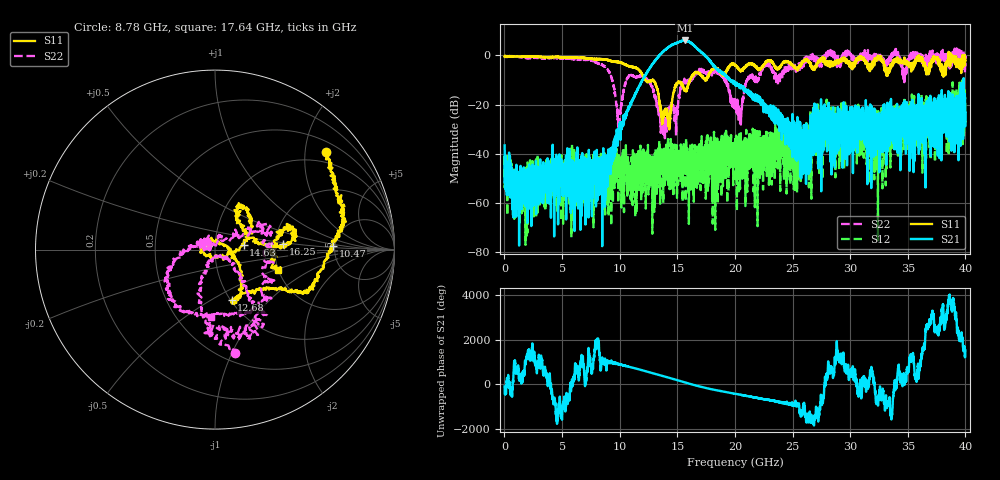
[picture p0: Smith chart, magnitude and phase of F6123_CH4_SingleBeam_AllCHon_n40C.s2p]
!Keysight Technologies,N5245B,MY55451909,A.17.20.08
!Date: Tuesday, November 21, 2023 17:28:04
!Correction: S11(C  2-Port  )
!S21(C  2-Port  )
!S12(C  2-Port  )
!S22(C  2-Port  )
!S2P File: Measurements: S11, S21, S12, S22:
# Hz S  RI  R 50
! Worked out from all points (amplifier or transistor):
!   4000 points, 10 MHz to 40 GHz, reference 50 ohm
!   highest |S21| = 6.1 dB at 15.64 GHz (marker M1)
!   |S21| within 3 dB of that: 14.18 GHz to 16.65 GHz (2.468 GHz wide, 16 % of centre)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
!   unconditionally stable (mu >= 1): start of sweep to 26.54 GHz; 26.75 GHz to 27.77 GHz; 32.61 GHz to 33.59 GHz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
!   at 6.67 GHz: K = 1996.61, MAG = -36.6 dB, |S12| = -46.4 dB
!   at 20.01 GHz: K = 145.94, MAG = -9.1 dB, |S12| = -42.6 dB
!   at 40 GHz: K = 23.65, MAG = -16.5 dB, |S12| = -23.7 dB
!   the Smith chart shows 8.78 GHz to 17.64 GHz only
!   S11 on the Smith chart (normalised r, x): 8.78 GHz: 0.74, +2.47; 10.47 GHz: 4.82, +0.38; 12.68 GHz: 1.01, -0.62; 14.63 GHz: 1.38, +0.08; 16.25 GHz: 2.21, +0.15; 17.64 GHz: 2.00, -0.53
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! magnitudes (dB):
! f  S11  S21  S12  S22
! 10 MHz  -0.4  -36.6  -41.1  -0.5
! 860 MHz  -0.4  -58.6  -62.6  -0.4
! 6.68 GHz  -0.9  -40.8  -46.9  -1.7
! 8.78 GHz  -1.7  -57.1  -48.1  -4.6
! 9.89 GHz  -2.7  -30.0  -42.7  -29.1
! 10.47 GHz  -3.6  -25.7  -45.9  -11.9
! 12.68 GHz  -10.6  -4.8  -47.5  -11.7
! 13.34 GHz  -15.3  -0.6  -45.5  -20.8
! 14.22 GHz  -28.8  3.3  -53.5  -25.8
! 14.63 GHz  -15.8  4.4  -48.0  -20.1
! 15.64 GHz  -13.9  6.1  -47.4  -9.8
! 16.25 GHz  -8.4  4.8  -43.0  -9.1
! 17.64 GHz  -8.6  -1.2  -42.1  -8.5
! 20.01 GHz  -3.8  -11.5  -42.6  -18.1
! 20.44 GHz  -6.1  -12.4  -54.4  -27.5
! 21.11 GHz  -3.7  -15.2  -43.6  -9.7
! 22.65 GHz  -2.8  -20.4  -36.0  -3.3
! 23.73 GHz  -4.9  -28.1  -46.0  -11.4
! 25.79 GHz  -3.0  -39.8  -37.6  -5.1
! 26.67 GHz  -4.6  -24.8  -34.8  -1.1
! 33.34 GHz  -6.2  -25.7  -32.8  -3.6
! 40 GHz  -1.7  -23.1  -23.7  -4.4
